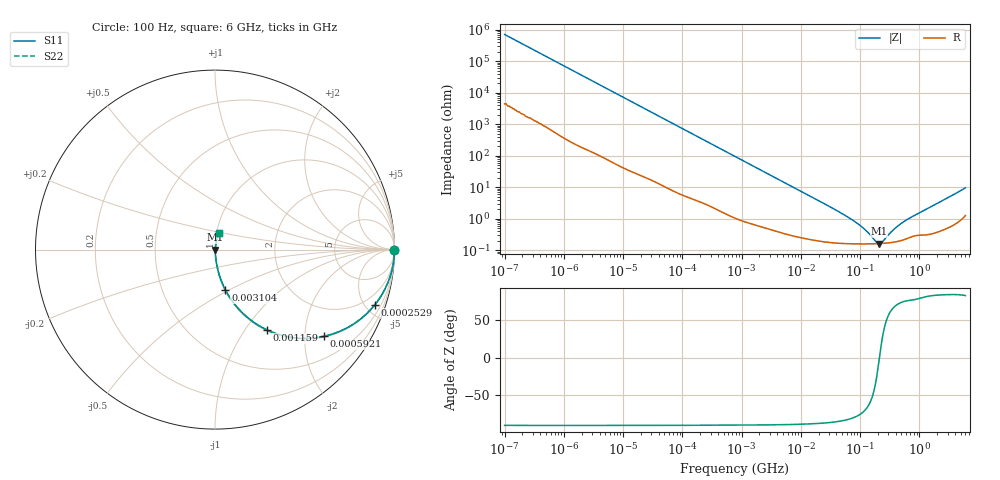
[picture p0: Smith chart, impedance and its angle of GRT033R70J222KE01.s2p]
!Murata Part Number: GRT033R70J222KE01
!These Parameters are Measured in Series Mode Connection
!Data Generated on Jun 19, 2026
!  o--ll--o
!Port1  Port2
!  o------o
!Operation Temp=25[degC], DC Bias Voltage=0[V]
!Freq. Start=100[Hz] Stop=6[GHz] 401[Steps]
# Hz S RI R 50
!Freq.(Hz) S11(Real) S11(Imag) S21(Real) S21(Imag) S12(Real) S12(Imag) S22(Real) S22(Imag)
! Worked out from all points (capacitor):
!   401 points, 100 Hz to 6 GHz, reference 50 ohm
!   read as one part in series: C = 2.24 nF near 109 Hz
!   lowest |Z| = 163 mohm at 208.8 MHz (marker M1)
!   series resonance near 212.3 MHz, so ESL is about 250 pH
!   S11 on the Smith chart (normalised r, x): 100 Hz: open; 252.9 kHz: 1.06, -5.79; 592.1 kHz: 1.03, -2.48; 1.159 MHz: 1.02, -1.27; 3.104 MHz: 1.01, -0.48; 6 GHz: 1.03, +0.19
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100  1 -0.000141  9e-07 0.000141  9e-07 0.000141  1 -0.000141
2008  1 -0.0028  2.22e-05 0.0028  2.22e-05 0.0028  1 -0.0028
40335  0.9965 -0.0554  0.00348 0.0554  0.00348 0.0554  0.9965 -0.0554
108014  0.9774 -0.1448  0.0226 0.1448  0.0226 0.1448  0.9774 -0.1448
252896  0.8909 -0.3069  0.1091 0.3069  0.1091 0.3069  0.8909 -0.3069
378399  0.7875 -0.404  0.2125 0.404  0.2125 0.404  0.7875 -0.404
592111  0.6058 -0.4835  0.3942 0.4835  0.3942 0.4835  0.6058 -0.4835
774597  0.4751 -0.4939  0.5249 0.4939  0.5249 0.4939  0.4751 -0.4939
1159002  0.2908 -0.448  0.7092 0.448  0.7092 0.448  0.2908 -0.448
1813585  0.1464 -0.3462  0.8536 0.3462  0.8536 0.3462  0.1464 -0.3462
3103719  0.058 -0.2246  0.942 0.2246  0.942 0.2246  0.058 -0.2246
6353432  0.0166 -0.1154  0.9834 0.1154  0.9834 0.1154  0.0166 -0.1154
1.555665e7  0.00442 -0.0479  0.9956 0.0479  0.9956 0.0479  0.00442 -0.0479
8.154455e7  0.00165 -0.00793  0.9984 0.00793  0.9984 0.00793  0.00165 -0.00793
1.166697e8  0.0016 -0.00454  0.9984 0.00454  0.9984 0.00454  0.0016 -0.00454
1.825626e8  0.00161 -0.00108  0.9984 0.00108  0.9984 0.00108  0.00161 -0.00108
2.088084e8  0.00162 -0.000118  0.9984 0.000118  0.9984 0.000118  0.00162 -0.000118
2.388273e8  0.00164 0.000843  0.9984 -0.000843  0.9984 -0.000843  0.00164 0.000843
3.124326e8  0.00172 0.00283  0.9983 -0.00283  0.9983 -0.00283  0.00172 0.00283
4.274388e8  0.00191 0.0054  0.9981 -0.0054  0.9981 -0.0054  0.00191 0.0054
6.395615e8  0.00247 0.00936  0.9975 -0.00936  0.9975 -0.00936  0.00247 0.00936
6e9  0.0211 0.0918  0.9789 -0.0918  0.9789 -0.0918  0.0211 0.0918
